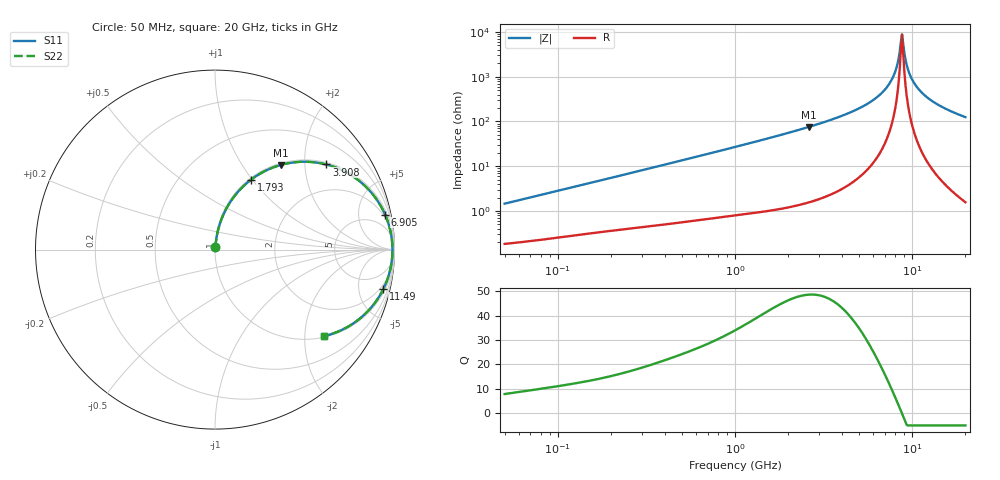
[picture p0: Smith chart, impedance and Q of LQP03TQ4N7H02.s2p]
!Murata Part Number: LQP03TQ4N7H02
!These Parameters are Measured in Series Mode Connection
!  o--[Z]--o
!Port1  Port2
!  o-------o
!Freq. Start=50[MHz] Stop=20[GHz], 401[Steps]
# Hz S RI R 50
!Freq.(Hz) S11(Real) S11(Imag) S21(Real) S21(Imag) S12(Real) S12(Imag) S22(Real) S22(Imag)
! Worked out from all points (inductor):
!   401 points, 50 MHz to 20 GHz, reference 50 ohm
!   read as one part in series: L = 4.56 nH near 51.52 MHz
!   highest Q = 48.6 at 2.608 GHz (marker M1), where L = 4.6 nH
!   self-resonance near 8.645 GHz
!   S11 on the Smith chart (normalised r, x): 50 MHz: 1.00, +0.03; 1.793 GHz: 1.02, +0.99; 3.908 GHz: 1.06, +2.57; 6.905 GHz: 1.56, +9.55; 11.49 GHz: 1.38, -8.40; 20 GHz: 1.03, -2.50
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5e7  0.00204 0.0144  0.998 -0.0144  0.998 -0.0144  0.00204 0.0144
1.364002e8  0.00441 0.0377  0.9956 -0.0377  0.9956 -0.0377  0.00441 0.0377
3.721004e8  0.0147 0.0988  0.9853 -0.0988  0.9853 -0.0988  0.0147 0.0988
1e9  0.0739 0.2473  0.9261 -0.2473  0.9261 -0.2473  0.0739 0.2473
1.793498e9  0.2018 0.3903  0.7982 -0.3903  0.7982 -0.3903  0.2018 0.3903
2.608132e9  0.3654 0.4714  0.6346 -0.4714  0.6346 -0.4714  0.3654 0.4714
2.728004e9  0.3902 0.4776  0.6098 -0.4776  0.6098 -0.4776  0.3902 0.4776
3.908127e9  0.62 0.4741  0.38 -0.4741  0.38 -0.4741  0.62 0.4741
5.515528e9  0.8443 0.3464  0.1557 -0.3464  0.1557 -0.3464  0.8443 0.3464
6.905011e9  0.9476 0.1954  0.0524 -0.1954  0.0524 -0.1954  0.9476 0.1954
7.442007e9  0.969 0.1365  0.031 -0.1365  0.031 -0.1365  0.969 0.1365
8.020766e9  0.9828 0.0749  0.0172 -0.0749  0.0172 -0.0749  0.9828 0.0749
8.264682e9  0.9861 0.0498  0.0139 -0.0498  0.0139 -0.0498  0.9861 0.0498
8.516016e9  0.9881 0.0245  0.0119 -0.0245  0.0119 -0.0245  0.9881 0.0245
8.774992e9  0.9888 -0.000905  0.0112 0.000905  0.0112 0.000905  0.9888 -0.000905
8.907419e9  0.9887 -0.0136  0.0113 0.0136  0.0113 0.0136  0.9887 -0.0136
9.316812e9  0.9863 -0.0516  0.0137 0.0516  0.0137 0.0516  0.9863 -0.0516
9.745021e9  0.981 -0.0892  0.019 0.0892  0.019 0.0892  0.981 -0.0892
1.050288e10  0.9658 -0.1506  0.0342 0.1506  0.0342 0.1506  0.9658 -0.1506
1.149051e10  0.9377 -0.2204  0.0623 0.2204  0.0623 0.2204  0.9377 -0.2204
1.460232e10  0.8187 -0.3743  0.1813 0.3743  0.1813 0.3743  0.8187 -0.3743
2e10  0.609 -0.4817  0.391 0.4817  0.391 0.4817  0.609 -0.4817
